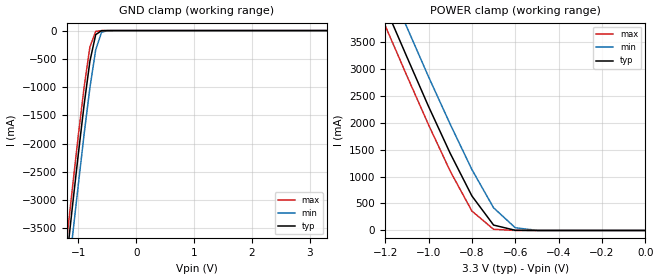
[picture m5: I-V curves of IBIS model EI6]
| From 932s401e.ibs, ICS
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|   Model EI6
[Model]   EI6
Model_type   Input
Vinl =   0.80V
Vinh =   2.00V
C_comp   2.50pF   2.00pF   3.00pF
[Temperature Range]   27.00   70.00   0.000
[Voltage Range]   3.30V   3.00V   3.70V
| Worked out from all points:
|   GND clamp passes 1 mA (typ) near -0.54 V on its own axis
|   POWER clamp passes 1 mA (typ) near -0.53 V on its own axis
[GND_clamp]
| voltage   I(typ)   I(min)   I(max)
-3.3V     -24.55A    -25.06A    -24.24A
-1.2V     -4.03A     -4.56A     -3.69A
-1.1V     -3.09A     -3.63A     -2.76A
-1V       -2.18A     -2.72A     -1.85A
-900mV    -1.31A     -1.83A     -1A
-800mV    -540mA     -1.01A     -290mA
-700mV    -71.73mA   -340mA     -14.36mA
-600mV    -2.26mA    -32.35mA   -430uA
-500mV    -85.82uA   -1.3mA     -27.2uA
3.3V      71.48pA    2.74uA     48.84pA
[POWER_clamp]
| voltage   I(typ)   I(min)   I(max)
-3.3V     24.69A     25.21A     24.37A
-1.2V     4.15A      4.71A      3.8A
-1.1V     3.22A      3.77A      2.87A
-1V       2.3A       2.85A      1.96A
-900mV    1.43A      1.97A      1.1A
-800mV    640mA      1.13A      360mA
-700mV    100mA      420mA      21.85mA
-600mV    3.35mA     50.51mA    380uA
-500mV    78.88uA    2.11mA     5.9uA
0V        71.48pA    320pA      74.52pA
